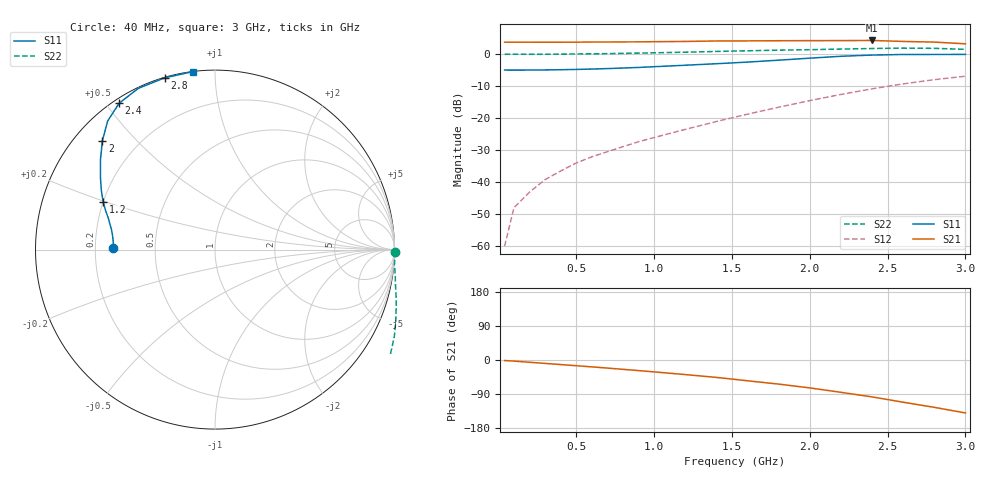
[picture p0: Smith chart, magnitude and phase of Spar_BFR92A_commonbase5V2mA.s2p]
! Filename:  BFR92ACA.S2P  Version:  2.0
! NXP part #: BFR92A  Date: Jul 1990
! Bias condition: Vce=5V, Ic=2mA
! COMMON BASE
#  MHz  S  MA  R  50
! Freq  S11  S21  S12  S22
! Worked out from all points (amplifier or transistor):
!   21 points, 40 MHz to 3 GHz, reference 50 ohm
!   highest |S21| = 4.3 dB at 2.4 GHz (marker M1)
!   |S21| within 3 dB of that: start of sweep to end of sweep
!   unconditionally stable (mu >= 1): nowhere
!   at 300 MHz: K = -0.22, MSG = 21.5 dB, |S12| = -39.2 dB
!   at 1 GHz: K = -0.80, MSG = 15.0 dB, |S12| = -26.0 dB
!   at 3 GHz: K = -0.46, MSG = 5.1 dB, |S12| = -6.8 dB
!   S11 on the Smith chart (normalised r, x): 40 MHz: 0.28, +0.01; 1.2 GHz: 0.20, +0.19; 2 GHz: 0.08, +0.40; 2.4 GHz: 0.02, +0.54; 2.8 GHz: 0.00, +0.75; 3 GHz: 0.00, +0.88
40  0.568 179.0  1.554 -1.4  0.001 72.2  1.002 -0.7
100  0.567 178.0  1.55 -2.9  0.004 86.0  1.005 -1.5
200  0.568 176.1  1.55 -6.0  0.007 94.8  1.003 -3.3
300  0.571 174.4  1.547 -9.0  0.011 99.8  1.003 -4.9
400  0.575 172.6  1.549 -12.0  0.015 104.5  1.009 -6.6
500  0.581 170.7  1.552 -15.1  0.02 106.8  1.015 -8.2
600  0.589 168.7  1.56 -18.1  0.025 110.9  1.02 -9.9
700  0.599 167.0  1.561 -21.3  0.03 114.0  1.027 -11.6
800  0.611 164.9  1.566 -24.6  0.036 116.8  1.036 -13.4
900  0.624 163.0  1.568 -27.9  0.043 119.5  1.047 -15.3
1000  0.641 161.1  1.579 -31.4  0.05 121.6  1.057 -17.2
1200  0.676 157.1  1.592 -38.4  0.067 126.1  1.082 -21.4
1400  0.714 152.5  1.619 -45.9  0.089 127.6  1.11 -25.8
1600  0.757 147.5  1.624 -54.8  0.116 129.2  1.138 -30.8
1800  0.811 141.9  1.634 -63.6  0.149 128.4  1.163 -36.6
2000  0.872 136.0  1.64 -73.6  0.189 126.5  1.184 -43.5
2200  0.933 129.9  1.642 -85.3  0.236 123.5  1.209 -51.5
2400  0.975 123.2  1.65 -97.3  0.289 119.1  1.234 -60.2
2600  0.995 115.4  1.592 -111.4  0.345 114.2  1.251 -68.9
2800  0.997 106.3  1.556 -124.9  0.402 108.0  1.243 -77.4
3000  0.999 97.2  1.462 -139.7  0.455 102.1  1.198 -86.2
